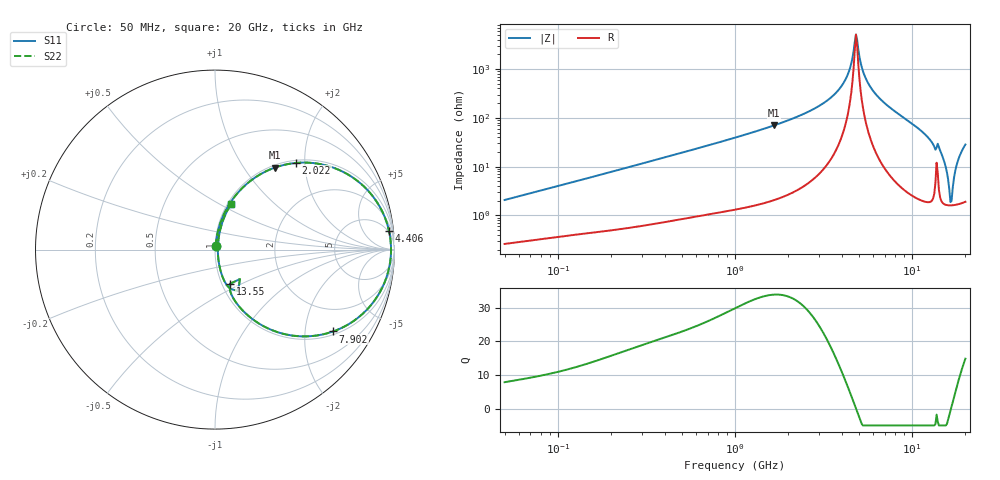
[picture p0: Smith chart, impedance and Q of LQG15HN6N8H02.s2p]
!Murata Part Number: LQG15HN6N8H02
!These Parameters are Measured in Series Mode Connection
!  o--[Z]--o
!Port1  Port2
!  o-------o
!Freq. Start=50[MHz] Stop=20[GHz], 401[Steps]
# Hz S RI R 50
!Freq.(Hz) S11(Real) S11(Imag) S21(Real) S21(Imag) S12(Real) S12(Imag) S22(Real) S22(Imag)
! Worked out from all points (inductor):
!   401 points, 50 MHz to 20 GHz, reference 50 ohm
!   read as one part in series: L = 6.47 nH near 51.52 MHz
!   highest Q = 33.9 at 1.664 GHz (marker M1), where L = 6.7 nH
!   self-resonance near 4.82 GHz
!   S11 on the Smith chart (normalised r, x): 50 MHz: 1.01, +0.04; 2.022 GHz: 1.05, +1.81; 4.406 GHz: 4, +18; 7.902 GHz: 1.10, -2.80; 13.55 GHz: 1.09, -0.43; 20 GHz: 1.04, +0.57
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5e7  0.00302 0.0204  0.997 -0.0204  0.997 -0.0204  0.00302 0.0204
1.364002e8  0.007 0.0532  0.993 -0.0532  0.993 -0.0532  0.007 0.0532
3.721004e8  0.0267 0.1388  0.9733 -0.1388  0.9733 -0.1388  0.0267 0.1388
1e9  0.1413 0.332  0.8587 -0.332  0.8587 -0.332  0.1413 0.332
1.664083e9  0.3338 0.4571  0.6662 -0.4571  0.6662 -0.4571  0.3338 0.4571
2.021818e9  0.4515 0.4828  0.5485 -0.4828  0.5485 -0.4828  0.4515 0.4828
2.728004e9  0.675 0.4506  0.325 -0.4506  0.325 -0.4506  0.675 0.4506
3.736399e9  0.9016 0.2658  0.0984 -0.2658  0.0984 -0.2658  0.9016 0.2658
4.405649e9  0.9698 0.1032  0.0302 -0.1032  0.0302 -0.1032  0.9698 0.1032
4.81993e9  0.9809 0.00207  0.0191 -0.00207  0.0191 -0.00207  0.9809 0.00207
5.273168e9  0.9699 -0.1021  0.0301 0.1021  0.0301 0.1021  0.9699 -0.1021
5.598765e9  0.9498 -0.1704  0.0502 0.1704  0.0502 0.1704  0.9498 -0.1704
7.442007e9  0.7252 -0.4265  0.2748 0.4265  0.2748 0.4265  0.7252 -0.4265
7.901521e9  0.6574 -0.4563  0.3426 0.4563  0.3426 0.4563  0.6574 -0.4563
1.034674e10  0.329 -0.4531  0.671 0.4531  0.671 0.4531  0.329 -0.4531
1.354865e10  0.0844 -0.1899  0.9156 0.1899  0.9156 0.1899  0.0844 -0.1899
1.438523e10  0.0646 -0.1968  0.9354 0.1968  0.9354 0.1968  0.0646 -0.1968
1.504638e10  0.0353 -0.1325  0.9647 0.1325  0.9647 0.1325  0.0353 -0.1325
1.646126e10  0.0159 -0.00945  0.9841 0.00945  0.9841 0.00945  0.0159 -0.00945
1.696185e10  0.017 0.0318  0.983 -0.0318  0.983 -0.0318  0.017 0.0318
1.828096e10  0.0355 0.1347  0.9645 -0.1347  0.9645 -0.1347  0.0355 0.1347
2e10  0.0891 0.2532  0.9109 -0.2532  0.9109 -0.2532  0.0891 0.2532
